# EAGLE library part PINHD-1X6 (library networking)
PIN HEADER
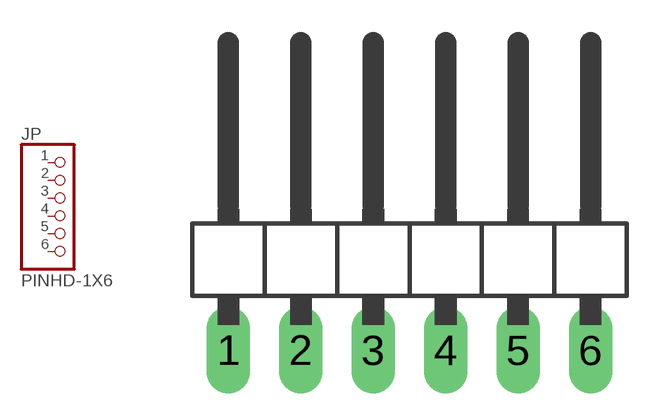
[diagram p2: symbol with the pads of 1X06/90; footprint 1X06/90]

Designator prefix JP

## PINHD-1X6/90  [1X06/90]
1  1  pas
2  2  pas
3  3  pas
4  4  pas
5  5  pas
6  6  pas

## Footprint 1X06/90 (pad centres in mm)
PIN HEADER
drill 1.016 long: 1 -6.35,-3.81; 2 -3.81,-3.81; 3 -1.27,-3.81; 4 1.27,-3.81; 5 3.81,-3.81; 6 6.35,-3.81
